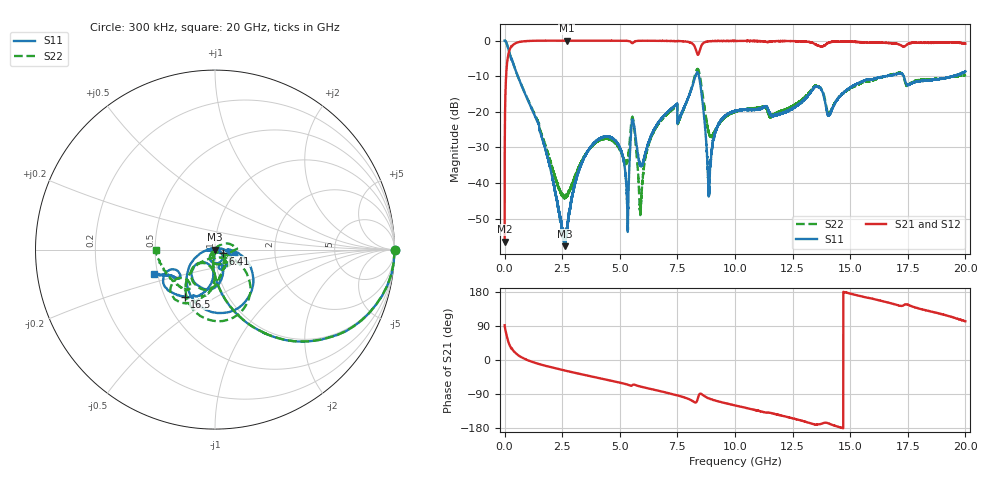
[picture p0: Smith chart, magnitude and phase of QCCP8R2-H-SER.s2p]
!QCCP8R2
!Johanson Technology Inc.
!www.johansontechnology.com
!Test Board Conditions:
!Substrate Type  RO4350B
!Substrate Thickness  20 mil
!Substrate Dk  3.66
!TL Type: GCPW
!TL Trace Width  36 mil
!TL Gap  12 mil
!Electrode orientation  Horizontal
!DUT TOPOLOGY	SERIES
!Mounting Pad LxW  26x36 mil
# MHz S  dB  R 50
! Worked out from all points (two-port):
!   20001 points, 300 kHz to 20 GHz, reference 50 ohm
!   highest |S21| = -0.02 dB at 2.699 GHz (marker M1); lowest = -56.4 dB at 300 kHz (marker M2)
!   |S21| within 3 dB of the highest: 194.5 MHz to 8.325 GHz (8.131 GHz wide, 191 % of centre); 8.459 GHz to end of sweep
!   lowest |S11| = -57.7 dB at 2.624 GHz (marker M3), VSWR 1.00, Z = 49.9 - j0.12 ohm
!   |S11| at or under -10 dB: 571.6 MHz to 8.281 GHz (7.71 GHz wide, 174 % of centre); 8.437 GHz to 16.53 GHz (8.088 GHz wide, 64.8 % of centre); 17.32 GHz to 19.46 GHz (2.139 GHz wide, 11.6 % of centre)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
!   |S22| runs from -49.0 to 0.0 dB; largest |S21 - S12| = 0.037
!   S11 on the Smith chart (normalised r, x): 300 kHz: open; 6.41 GHz: 1.09, -0.05; 16.5 GHz: 0.63, -0.36; 20 GHz: 0.48, -0.15
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0.3  0.00 -0.2  -56.40 91.6  -56.44 88.8  0.00 -0.1
108.298  -1.17 -30.0  -6.28 59.6  -6.30 59.7  -1.18 -30.1
260.296  -4.56 -55.6  -1.95 33.7  -1.94 33.8  -4.58 -55.6
2624.261  -57.69 -112.6  -0.04 -28.0  -0.04 -27.9  -43.85 -128.4
2699.26  -52.96 -134.7  -0.03 -29.0  -0.04 -29.0  -43.49 -121.2
3334.25  -34.63 -163.2  -0.04 -37.7  -0.04 -37.6  -34.08 -99.3
4645.23  -27.32 179.9  -0.06 -55.0  -0.04 -55.0  -27.99 -103.7
5318.22  -45.82 138.4  -0.09 -64.7  -0.08 -64.7  -33.91 -49.4
5558.217  -22.29 -83.0  -0.73 -65.8  -0.73 -65.9  -21.57 -79.6
5905.211  -35.24 -91.6  -0.08 -70.2  -0.07 -70.2  -47.38 110.9
6410.204  -25.92 -25.2  -0.09 -77.4  -0.09 -77.5  -26.43 38.0
6667.2  -23.07 -20.8  -0.08 -81.0  -0.10 -81.1  -23.46 30.9
7600.186  -21.54 -0.8  -0.15 -95.1  -0.15 -95.0  -21.97 -25.6
8376.174  -8.98 -84.1  -3.95 -103.9  -3.96 -104.1  -7.96 -85.4
8882.167  -42.20 52.4  -0.22 -101.4  -0.22 -101.6  -26.14 -106.2
9222.162  -24.44 -3.5  -0.15 -108.3  -0.14 -108.5  -24.47 -48.3
10000.15  -19.69 -32.3  -0.11 -119.8  -0.12 -119.8  -20.05 -30.3
13334.1  -14.07 -85.3  -0.58 -168.2  -0.58 -168.3  -13.68 -92.0
14090.09  -20.86 -114.0  -0.55 -168.1  -0.56 -168.2  -20.56 -112.3
16499.05  -10.12 -122.9  -0.63 153.9  -0.58 153.6  -10.04 -111.8
16667.05  -9.91 -126.6  -0.70 151.2  -0.61 150.6  -9.74 -114.0
20000  -8.68 -157.9  -0.87 102.4  -0.75 103.8  -9.66 -179.6
